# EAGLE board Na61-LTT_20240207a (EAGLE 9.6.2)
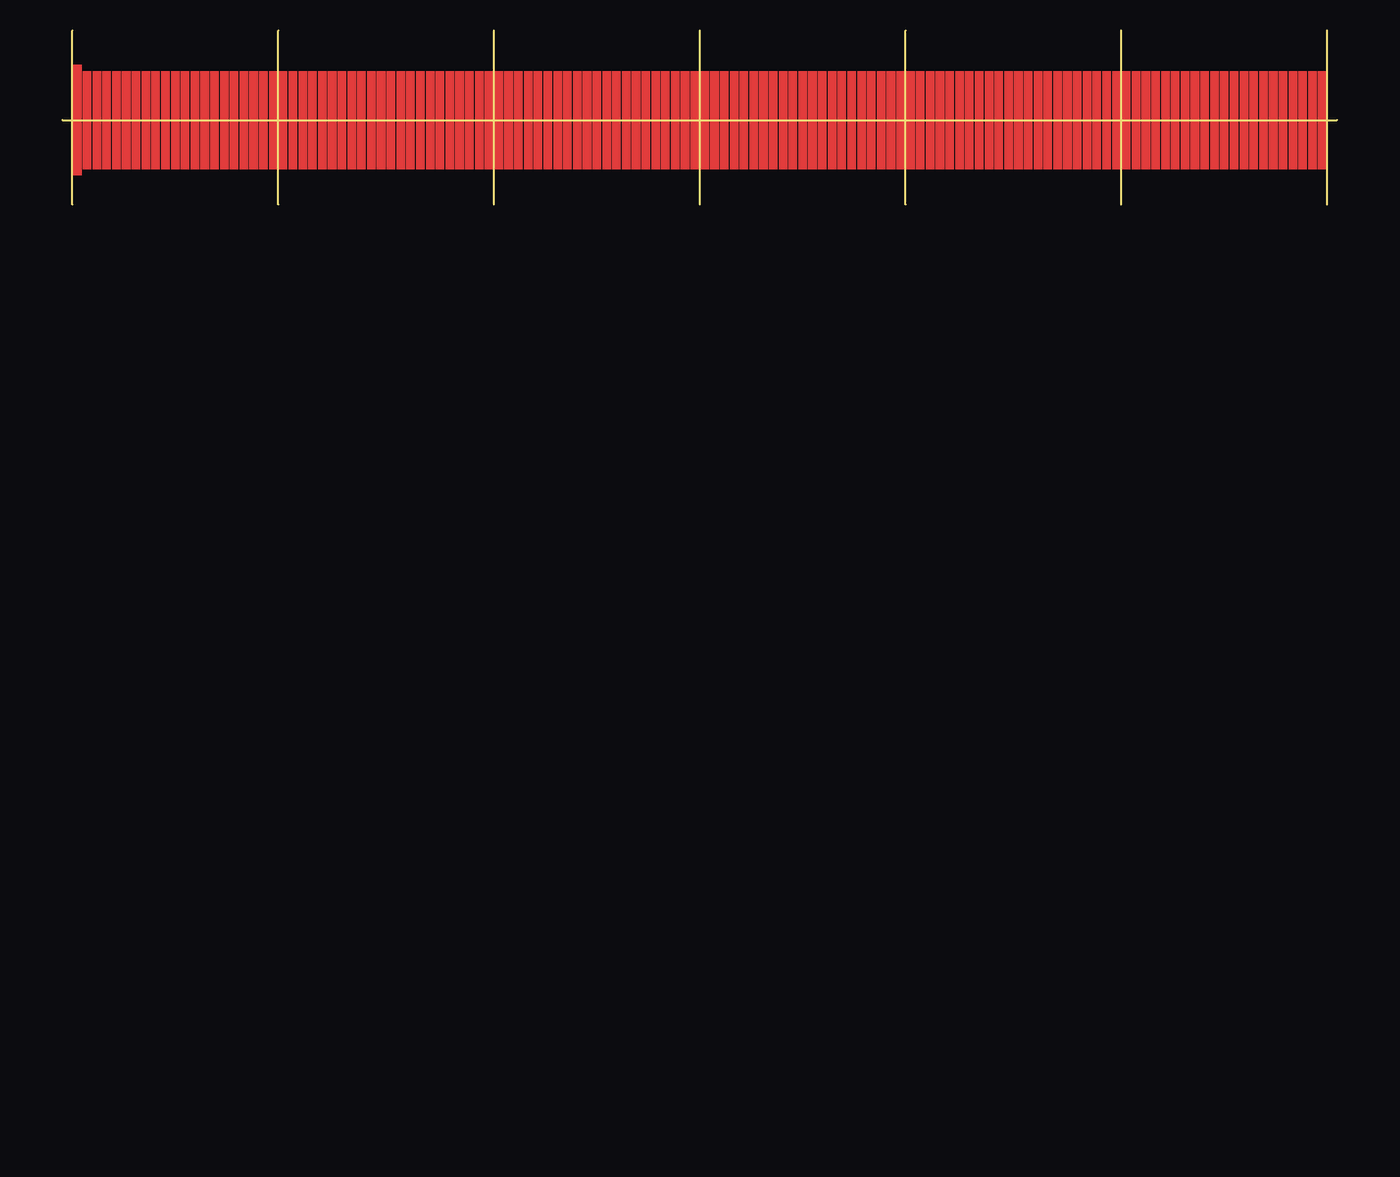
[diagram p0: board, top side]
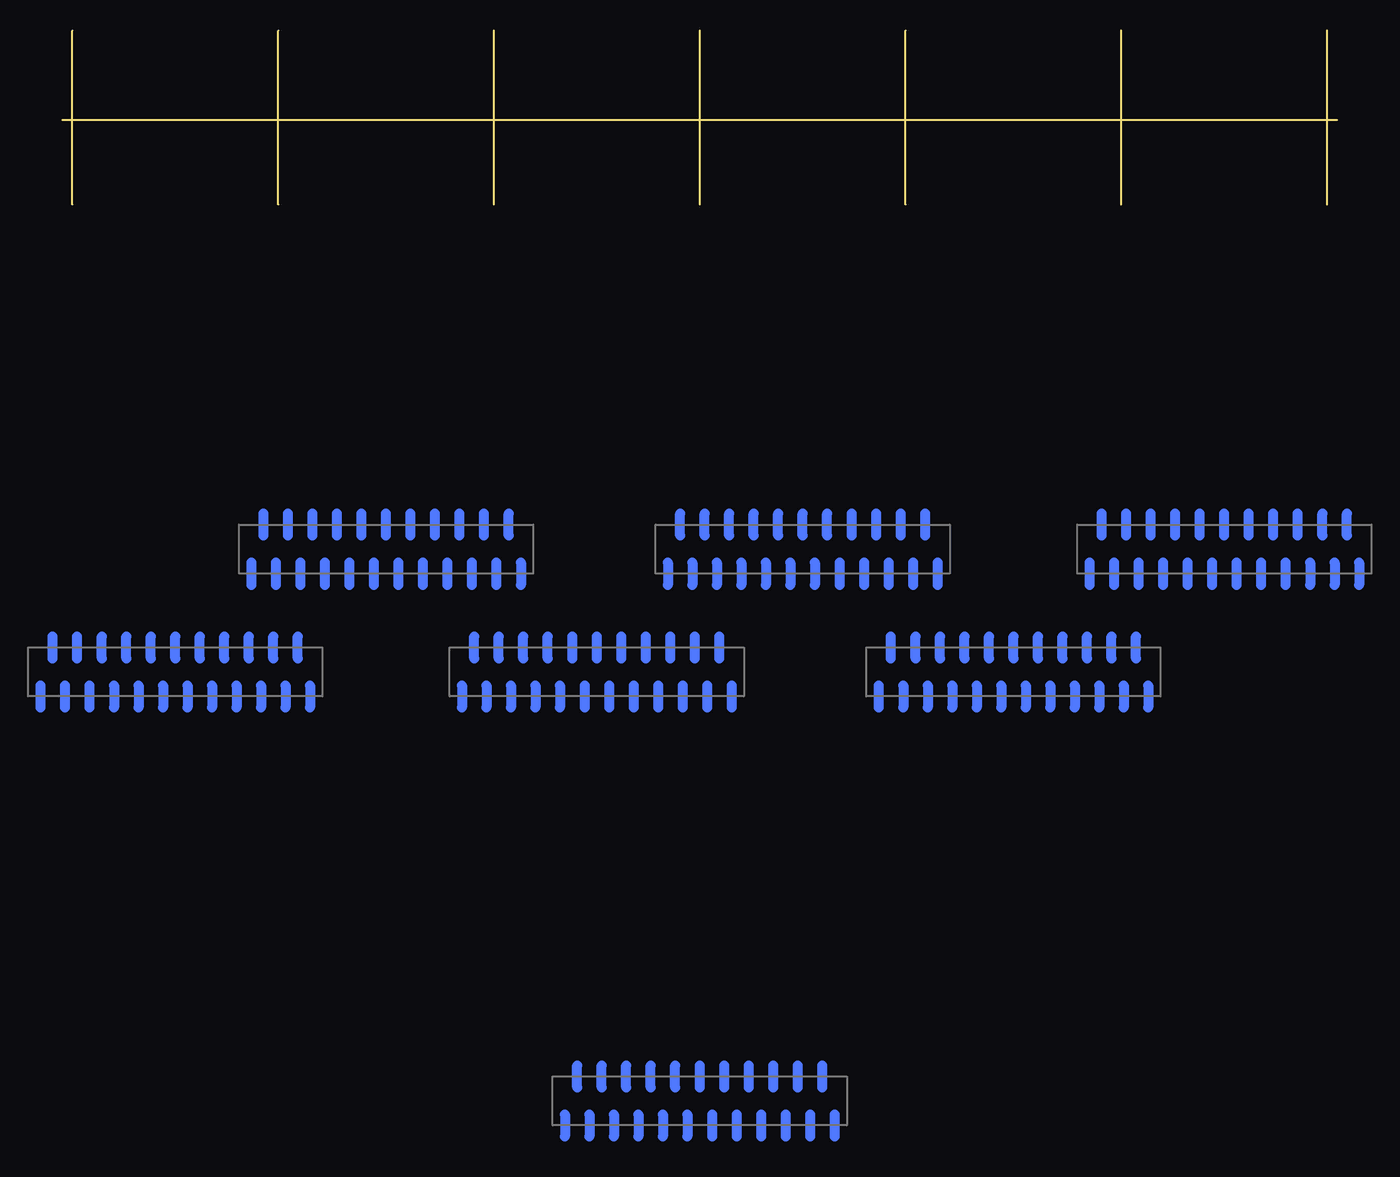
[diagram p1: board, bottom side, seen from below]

Size 104 x 14.2 mm. Coordinates in mm from the lower left corner, seen from the top.
Outline: 52,0 52,14.2
Outline: 35.2,0 35.2,14.2
Outline: 17.6,0 17.6,14.2
Outline: 0.8,0 0.8,14.2
Outline: 68.8,0 68.8,14.2
Outline: 86.4,0 86.4,14.2
Outline: 103.2,0 103.2,14.2
Outline: 0,6.9 104,6.9
Copper layers (1*16): Top 0.035mm / dielectric 1.5mm / Bottom 0.035mm
Design rules "default *": minimum track width 6mil, minimum drill 0.2mm, track to track 6mil, track to pad 6mil, pad to pad 6mil, via to via 6mil, smd to smd 6mil, copper to edge 40mil, drill to drill 6mil, minimum pad ring 8mil, minimum via ring 4mil, stop-mask expansion 4mil, vias tented up to drill 0mil, thermal gap 10mil

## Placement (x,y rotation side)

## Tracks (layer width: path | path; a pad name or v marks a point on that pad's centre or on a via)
S$1
  Bottom 0.8: 63.4,-39.2 63.4,-41
S$2
  Bottom 0.8: 62.4,-37 62.4,-35.2
S$3
  Bottom 0.8: 59.4,-39.2 59.4,-41
S$4
  Bottom 0.8: 56.4,-37 56.4,-35.2
S$5
  Bottom 0.8: 53.4,-39.2 53.4,-41
S$6
  Bottom 0.8: 52.4,-37 52.4,-35.2
S$7
  Bottom 0.8: 49.4,-39.2 49.4,-41
S$8
  Bottom 0.8: 50.4,-37 50.4,-35.2
S$9
  Bottom 0.8: 71.4,-39.2 71.4,-41
S$10
  Bottom 0.8: 70.4,-37 70.4,-35.2
S$11
  Bottom 0.8: 67.4,-39.2 67.4,-41
S$12
  Bottom 0.8: 66.4,-37 66.4,-35.2
S$13
  Bottom 0.8: 68.4,-37 68.4,-35.2
S$14
  Bottom 0.8: 69.4,-39.2 69.4,-41
S$15
  Bottom 0.8: 65.4,-39.2 65.4,-41
S$16
  Bottom 0.8: 64.4,-37 64.4,-35.2
S$17
  Bottom 0.8: 60.4,-37 60.4,-35.2
S$18
  Bottom 0.8: 61.4,-39.2 61.4,-41
S$19
  Bottom 0.8: 57.4,-39.2 57.4,-41
S$20
  Bottom 0.8: 58.4,-37 58.4,-35.2
S$21
  Bottom 0.8: 54.4,-37 54.4,-35.2
S$22
  Bottom 0.8: 55.4,-39.2 55.4,-41
S$23
  Bottom 0.8: 51.4,-39.2 51.4,-41
S$24
  Bottom 0.8: 44.6,-29.2 44.6,-31
S$25
  Bottom 0.8: 46.6,-29.2 46.6,-31
S$26
  Bottom 0.8: 43.6,-27 43.6,-25.2
S$27
  Bottom 0.8: 45.6,-27 45.6,-25.2
S$28
  Bottom 0.8: 40.6,-29.2 40.6,-31
S$29
  Bottom 0.8: 42.6,-29.2 42.6,-31
S$30
  Bottom 0.8: 41.6,-27 41.6,-25.2
S$31
  Bottom 0.8: 39.6,-27 39.6,-25.2
S$32
  Bottom 0.8: 38.6,-29.2 38.6,-31
S$33
  Bottom 0.8: 36.6,-29.2 36.6,-31
S$34
  Bottom 0.8: 37.6,-27 37.6,-25.2
S$35
  Bottom 0.8: 35.6,-27 35.6,-25.2
S$36
  Bottom 0.8: 34.6,-29.2 34.6,-31
S$37
  Bottom 0.8: 32.6,-29.2 32.6,-31
S$38
  Bottom 0.8: 33.6,-27 33.6,-25.2
S$39
  Bottom 0.8: 52.6,-29.2 52.6,-31
S$40
  Bottom 0.8: 54.6,-29.2 54.6,-31
S$41
  Bottom 0.8: 51.6,-27 51.6,-25.2
S$42
  Bottom 0.8: 53.6,-27 53.6,-25.2
S$43
  Bottom 0.8: 48.6,-29.2 48.6,-31
S$44
  Bottom 0.8: 50.6,-29.2 50.6,-31
S$45
  Bottom 0.8: 47.6,-27 47.6,-25.2
S$46
  Bottom 0.8: 49.6,-27 49.6,-25.2
S$47
  Bottom 0.8: 27.4,-39.2 27.4,-41
S$48
  Bottom 0.8: 29.4,-39.2 29.4,-41
S$49
  Bottom 0.8: 26.4,-37 26.4,-35.2
S$50
  Bottom 0.8: 28.4,-37 28.4,-35.2
S$51
  Bottom 0.8: 23.4,-39.2 23.4,-41
S$52
  Bottom 0.8: 25.4,-39.2 25.4,-41
S$53
  Bottom 0.8: 24.4,-37 24.4,-35.2
S$54
  Bottom 0.8: 22.4,-37 22.4,-35.2
S$55
  Bottom 0.8: 21.4,-39.2 21.4,-41
S$56
  Bottom 0.8: 19.4,-39.2 19.4,-41
S$57
  Bottom 0.8: 20.4,-37 20.4,-35.2
S$58
  Bottom 0.8: 18.4,-37 18.4,-35.2
S$59
  Bottom 0.8: 17.4,-39.2 17.4,-41
S$60
  Bottom 0.8: 15.4,-39.2 15.4,-41
S$61
  Bottom 0.8: 16.4,-37 16.4,-35.2
S$62
  Bottom 0.8: 35.4,-39.2 35.4,-41
S$63
  Bottom 0.8: 37.4,-39.2 37.4,-41
S$64
  Bottom 0.8: 34.4,-37 34.4,-35.2
S$65
  Bottom 0.8: 36.4,-37 36.4,-35.2
S$66
  Bottom 0.8: 31.4,-39.2 31.4,-41
S$67
  Bottom 0.8: 33.4,-39.2 33.4,-41
S$68
  Bottom 0.8: 30.4,-37 30.4,-35.2
S$69
  Bottom 0.8: 32.4,-37 32.4,-35.2
S$70
  Bottom 0.8: 78.6,-29.2 78.6,-31
S$71
  Bottom 0.8: 80.6,-29.2 80.6,-31
S$72
  Bottom 0.8: 77.6,-27 77.6,-25.2
S$73
  Bottom 0.8: 79.6,-27 79.6,-25.2
S$74
  Bottom 0.8: 74.6,-29.2 74.6,-31
S$75
  Bottom 0.8: 76.6,-29.2 76.6,-31
S$76
  Bottom 0.8: 75.6,-27 75.6,-25.2
S$77
  Bottom 0.8: 73.6,-27 73.6,-25.2
S$78
  Bottom 0.8: 72.6,-29.2 72.6,-31
S$79
  Bottom 0.8: 70.6,-29.2 70.6,-31
S$80
  Bottom 0.8: 71.6,-27 71.6,-25.2
S$81
  Bottom 0.8: 69.6,-27 69.6,-25.2
S$82
  Bottom 0.8: 68.6,-29.2 68.6,-31
S$83
  Bottom 0.8: 66.6,-29.2 66.6,-31
S$84
  Bottom 0.8: 67.6,-27 67.6,-25.2
S$85
  Bottom 0.8: 86.6,-29.2 86.6,-31
S$86
  Bottom 0.8: 88.6,-29.2 88.6,-31
S$87
  Bottom 0.8: 85.6,-27 85.6,-25.2
S$88
  Bottom 0.8: 87.6,-27 87.6,-25.2
S$89
  Bottom 0.8: 82.6,-29.2 82.6,-31
S$90
  Bottom 0.8: 84.6,-29.2 84.6,-31
S$91
  Bottom 0.8: 81.6,-27 81.6,-25.2
S$92
  Bottom 0.8: 83.6,-27 83.6,-25.2
S$93
  Bottom 0.8: 10.2,-29.2 10.2,-31
S$94
  Bottom 0.8: 12.2,-29.2 12.2,-31
S$95
  Bottom 0.8: 9.2,-27 9.2,-25.2
S$96
  Bottom 0.8: 11.2,-27 11.2,-25.2
S$97
  Bottom 0.8: 6.2,-29.2 6.2,-31
S$98
  Bottom 0.8: 8.2,-29.2 8.2,-31
S$99
  Bottom 0.8: 7.2,-27 7.2,-25.2
S$100
  Bottom 0.8: 5.2,-27 5.2,-25.2
S$101
  Bottom 0.8: 4.2,-29.2 4.2,-31
S$102
  Bottom 0.8: 2.2,-29.2 2.2,-31
S$103
  Bottom 0.8: 3.2,-27 3.2,-25.2
S$104
  Bottom 0.8: 1.2,-27 1.2,-25.2
S$105
  Bottom 0.8: 0.2,-29.2 0.2,-31
S$106
  Bottom 0.8: -1.8,-29.2 -1.8,-31
S$107
  Bottom 0.8: -0.8,-27 -0.8,-25.2
S$108
  Bottom 0.8: 18.2,-29.2 18.2,-31
S$109
  Bottom 0.8: 20.2,-29.2 20.2,-31
S$110
  Bottom 0.8: 17.2,-27 17.2,-25.2
S$111
  Bottom 0.8: 19.2,-27 19.2,-25.2
S$112
  Bottom 0.8: 14.2,-29.2 14.2,-31
S$113
  Bottom 0.8: 16.2,-29.2 16.2,-31
S$114
  Bottom 0.8: 13.2,-27 13.2,-25.2
S$115
  Bottom 0.8: 15.2,-27 15.2,-25.2
S$116
  Bottom 0.8: 95.8,-39.2 95.8,-41
S$117
  Bottom 0.8: 97.8,-39.2 97.8,-41
S$118
  Bottom 0.8: 94.8,-37 94.8,-35.2
S$119
  Bottom 0.8: 96.8,-37 96.8,-35.2
S$120
  Bottom 0.8: 91.8,-39.2 91.8,-41
S$121
  Bottom 0.8: 93.8,-39.2 93.8,-41
S$122
  Bottom 0.8: 92.8,-37 92.8,-35.2
S$123
  Bottom 0.8: 90.8,-37 90.8,-35.2
S$124
  Bottom 0.8: 89.8,-39.2 89.8,-41
S$125
  Bottom 0.8: 87.8,-39.2 87.8,-41
S$126
  Bottom 0.8: 88.8,-37 88.8,-35.2
S$127
  Bottom 0.8: 86.8,-37 86.8,-35.2
S$128
  Bottom 0.8: 85.8,-39.2 85.8,-41
S$129
  Bottom 0.8: 83.8,-39.2 83.8,-41
S$130
  Bottom 0.8: 84.8,-37 84.8,-35.2
S$131
  Bottom 0.8: 103.8,-39.2 103.8,-41
S$132
  Bottom 0.8: 105.8,-39.2 105.8,-41
S$133
  Bottom 0.8: 102.8,-37 102.8,-35.2
S$134
  Bottom 0.8: 104.8,-37 104.8,-35.2
S$135
  Bottom 0.8: 99.8,-39.2 99.8,-41
S$136
  Bottom 0.8: 101.8,-39.2 101.8,-41
S$137
  Bottom 0.8: 98.8,-37 98.8,-35.2
S$138
  Bottom 0.8: 100.8,-37 100.8,-35.2
S$139
  Bottom 0.8: 53,-74.2 53,-76
S$140
  Bottom 0.8: 55,-74.2 55,-76
S$141
  Bottom 0.8: 52,-72 52,-70.2
S$142
  Bottom 0.8: 54,-72 54,-70.2
S$143
  Bottom 0.8: 49,-74.2 49,-76
S$144
  Bottom 0.8: 51,-74.2 51,-76
S$145
  Bottom 0.8: 50,-72 50,-70.2
S$146
  Bottom 0.8: 48,-72 48,-70.2
S$147
  Bottom 0.8: 47,-74.2 47,-76
S$148
  Bottom 0.8: 45,-74.2 45,-76
S$149
  Bottom 0.8: 46,-72 46,-70.2
S$150
  Bottom 0.8: 44,-72 44,-70.2
S$151
  Bottom 0.8: 43,-74.2 43,-76
S$152
  Bottom 0.8: 41,-74.2 41,-76
S$153
  Bottom 0.8: 42,-72 42,-70.2
S$154
  Bottom 0.8: 61,-74.2 61,-76
S$155
  Bottom 0.8: 63,-74.2 63,-76
S$156
  Bottom 0.8: 60,-72 60,-70.2
S$157
  Bottom 0.8: 62,-72 62,-70.2
S$158
  Bottom 0.8: 57,-74.2 57,-76
S$159
  Bottom 0.8: 59,-74.2 59,-76
S$160
  Bottom 0.8: 56,-72 56,-70.2
S$161
  Bottom 0.8: 58,-72 58,-70.2
(copper drawn outside any net)
  shapes: Top area x128

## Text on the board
Dimension: 00.0 / - 08.4 / 16.8 / - 25.6 / 34.4 / - 42.8 / 51.2
ConnRoute: Pad: 0.8 x 8 / VIA: szélén szélére, belül pont középre / PadRaw távolság : 8mm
